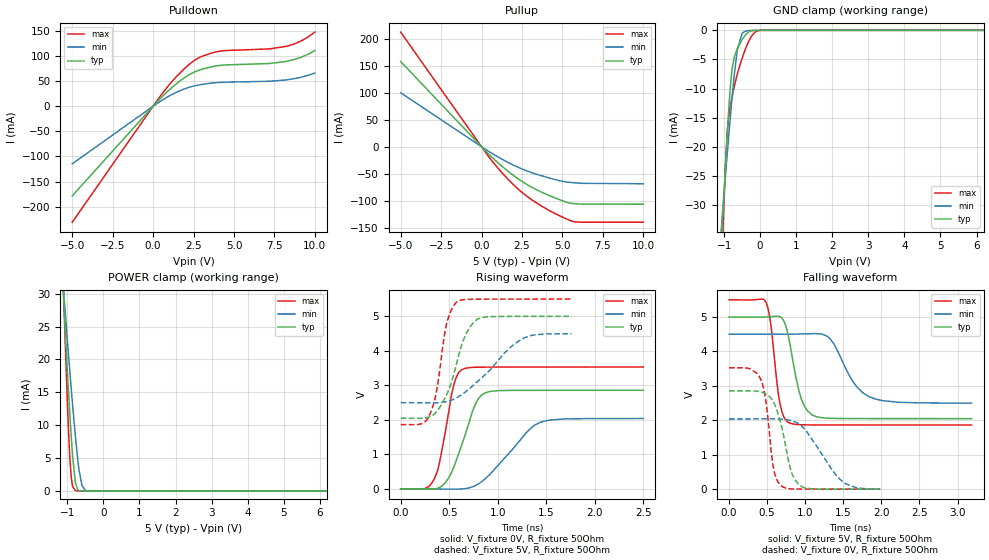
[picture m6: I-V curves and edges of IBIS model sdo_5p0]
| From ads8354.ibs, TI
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|   sdo_5p0 Model
[Model]   sdo_5p0
Model_type   3-state
Polarity   Non-Inverting
Vmeas = 2.5
Vref = 0
Cref = 10pF
Rref = 100
|   typ   min   max
|   (nom PVT)   (fast PVT)   (slow PVT)
C_comp   1.073e-12   8.568e-13   1.316e-12
| Where nom  PVT is Nominal Process, 5V, 27C
|   Fast PVT is Strong Process,  5.5V, -40C
|   Slow PVT is Weak Process,   4.5V, 125C
[Voltage Range]   5   4.5   5.5
|Junction Temperature
[Temperature Range]   27   125   -40
[Pullup Reference]   5   4.5   5.5
[Pulldown Reference]   0   0   0
[Power Clamp Reference]   5   4.5   5.5
[GND Clamp Reference]   0   0   0
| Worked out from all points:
|   slope of the pulldown table from 0 to 0.75 V, typ, clamps not added: 29.7 ohm
|   slope of the pullup table from 0 to 0.75 V, typ, clamps not added: 33.3 ohm
|   GND clamp passes 1 mA (typ) near -0.44 V on its own axis
|   POWER clamp passes 1 mA (typ) near -0.76 V on its own axis
|   falling waveform, V_fixture 5V, R_fixture 50Ohm: 20-80 % time 164ps typ, 305ps min, 111ps max; typ from 5 V to 2.05 V
|   rising waveform, V_fixture 0V, R_fixture 50Ohm: 20-80 % time 207ps typ, 381ps min, 137ps max; typ from 0 V to 2.86 V
|   rising waveform, V_fixture 5V, R_fixture 50Ohm: 20-80 % time 204ps typ, 424ps min, 121ps max; typ from 2.05 V to 5 V
|   falling waveform, V_fixture 0V, R_fixture 50Ohm: 20-80 % time 179ps typ, 373ps min, 113ps max; typ from 2.85 V to 0 V
[Pulldown]
|   Voltage   I(typ)   I(min)   I(max)
-5V       -178.3mA   -114.5mA   -230.7mA
382mV     13.36mA    8.452mA    17.42mA
1.3V      41.16mA    25.5mA     54.06mA
2.24V     62.82mA    37.76mA    83.52mA
2.861V    71.97mA    42.5mA     96.93mA
3.933V    80.43mA    46.96mA    108.5mA
4.449V    82.03mA    47.76mA    110.6mA
7.154V    84.94mA    49.63mA    114mA
8.248V    89.23mA    52.44mA    119.3mA
9.16V     97.58mA    57.78mA    130mA
10V       110.7mA    66.02mA    147.5mA
[GND Clamp]
|   Voltage   I(typ)   I(min)   I(max)
-5V       -581.4mA   -378.5mA   -904.4mA
-1.071V   -36.27mA   -33.51mA   -41.57mA
-1.012V   -29.1mA    -28.86mA   -30.98mA
-957.5mV  -22.68mA   -24.59mA   -22.48mA
-909.5mV  -17.4mA    -20.93mA   -17.22mA
-787mV    -7.107mA   -12.08mA   -11.69mA
-635mV    -3.13mA    -3.325mA   -7.49mA
-500mV    -1.565mA   -508.4uA   -4.782mA
-429.5mV  -947.7uA   -209.1uA   -3.547mA
-204mV    -54.66uA   -6.628uA   -711.8uA
-500uV    0A         0A         0A
10V       0A         0A         0A
[Pullup]
|   Voltage   I(typ)   I(min)   I(max)
-5V       157.9mA    100.1mA    212.4mA
458.5mV   -14.16mA   -8.977mA   -19mA
1.079V    -31.49mA   -20.1mA    -41.94mA
1.649V    -45.77mA   -29.31mA   -60.65mA
2.645V    -67.09mA   -43.05mA   -88.19mA
3.36V     -79.11mA   -50.73mA   -103.5mA
4.11V     -89.47mA   -57.28mA   -117mA
5.255V    -103.1mA   -65.48mA   -133.9mA
5.753V    -105.7mA   -66.96mA   -139.4mA
10V       -106.6mA   -68.7mA    -139.9mA
[POWER Clamp]
|   Voltage   I(typ)   I(min)   I(max)
-5V       422mA      299.4mA    614.5mA
-1.18V    37.56mA    36.02mA    41.53mA
-996mV    17.8mA     22.65mA    12.8mA
-950mV    13.35mA    19.46mA    7.015mA
-924.5mV  11.02mA    17.71mA    4.438mA
-891.5mV  8.17mA     15.49mA    2.059mA
-858.5mV  5.601mA    13.32mA    796.5uA
-775mV    1.187mA    8.148mA    53.17uA
-675.5mV  45.59uA    3.145mA    1.891uA
-594.5mV  2.382uA    827.4uA    192.5nA
-464mV    33.33nA    27.78uA    69.63nA
10V       0A         0A         0A
[Ramp]
R_load = 50
|   typ   min   max
dV/dt_r   1.71484/2.06879e-10   1.22446/3.81368e-10   2.11902/1.36498e-10
dV/dt_f   1.77058/1.63502e-10   1.20113/3.01551e-10   2.18201/1.11036e-10
[Falling Waveform]
V_fixture = 5V
V_fixture_min = 4.5V
V_fixture_max = 5.5V
R_fixture = 50Ohm
|   Time   V(typ)   V(min)   V(max)
0s        5V         4.5V       5.5V
489ps     5.001V     4.5V       5.415V
550.5ps   5.012V     4.5V       4.751V
670.5ps   5.005V     4.498V     2.469V
778ps     4.463V     4.498V     1.94V
952ps     2.604V     4.509V     1.871V
1.126ns   2.123V     4.517V     1.865V
1.326ns   2.059V     4.368V     1.864V
1.83ns    2.05V      2.696V     1.864V
3.185ns   2.049V     2.498V     1.863V
[Rising Waveform]
V_fixture = 0V
V_fixture_min = 0V
V_fixture_max = 0V
R_fixture = 50Ohm
|   Time   V(typ)   V(min)   V(max)
0s        13.59uV    3.891uV    255.2uV
246.5ps   -3.976mV   518.3uV    10.71mV
345ps     -1.244mV   -373.5uV   287.1mV
400ps     42.26mV    -1.71mV    768.4mV
550.5ps   654.8mV    -5.124mV   3.046V
627.5ps   1.267V     360.5uV    3.451V
776ps     2.495V     106mV      3.525V
913ps     2.821V     405.8mV    3.529V
1.436ns   2.857V     1.927V     3.531V
2.498ns   2.858V     2.041V     3.532V
[Rising Waveform]
V_fixture = 5V
V_fixture_min = 4.5V
V_fixture_max = 5.5V
R_fixture = 50Ohm
|   Time   V(typ)   V(min)   V(max)
0s        2.049V     2.498V     1.863V
209.5ps   2.047V     2.497V     1.883V
293.5ps   2.084V     2.493V     2.114V
375ps     2.254V     2.495V     2.918V
477ps     2.753V     2.533V     4.828V
578.5ps   3.664V     2.644V     5.417V
680ps     4.527V     2.839V     5.489V
831.5ps   4.965V     3.211V     5.497V
1.272ns   4.999V     4.374V     5.499V
1.761ns   4.999V     4.498V     5.5V
[Falling Waveform]
V_fixture = 0V
V_fixture_min = 0V
V_fixture_max = 0V
R_fixture = 50Ohm
|   Time   V(typ)   V(min)   V(max)
0s        2.853V     2.038V     3.524V
271ps     2.855V     2.038V     3.499V
417ps     2.823V     2.039V     3.191V
484ps     2.766V     2.04V      2.556V
593.5ps   2.489V     2.041V     504.2mV
690ps     1.823V     2.031V     92.08mV
815.5ps   520.4mV    1.989V     8.803mV
954.5ps   76.81mV    1.832V     2.899mV
1.481ns   1.149mV    237.3mV    1.019mV
1.985ns   29.92uV    81.19uV    257.5uV
